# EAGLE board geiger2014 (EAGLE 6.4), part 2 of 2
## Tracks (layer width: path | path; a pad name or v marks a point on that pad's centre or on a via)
N$1  (via drill 0.6)
  Top 0.406: v139.7,58.17 138.68,58.29 121.79,58.29 114.3,65.66 95.89,65.66 95.89,67.82 73.15,67.82 73.15,60.07 72.64,59.82 69.47,59.82 68.2,61.72 v55.24,61.72 | v55.24,56.26 55.24,30.61 54.61,29.97 33.27,29.97
  Top 0.61: v17.78,29.97 v21.97,29.97 33.27,29.97
  Top 0.813: v139.7,58.17 143,58.17 143,53.09 143.26,52.83 156.97,52.83 159.26,52.83 161.54,50.55 v161.42,50.44
  Top 1.016: v146.05,75.95 v146.05,74.93 v146.05,73.91 146.05,67.94 158.5,67.94 158.5,66.04 159.77,64.77 159.77,60.45 156.97,57.66 156.97,52.83
  Bottom 0.61: IC5.7 178.31,50.04 177.04,51.31 176.02,51.56 175.81,51.78 C19.+ | IC2.14 18.41,6.73 20.45,8.26 20.45,15.37 21.97,17.4 v21.97,29.97 | v17.78,29.97 T1.3 | v55.24,56.26 v55.24,61.72
  Bottom 0.813: IC4.14 160.02,49.02 160.02,50.44 v161.42,50.44 163.35,50.44 163.32,50.42 163.32,52.83 165.61,55.12 171.25,55.12 R38.1 174.23,54.91 C19.+ | Q4.3 v139.7,58.17
  Bottom 1.016: C13.1 147.06,79.5 147.32,79.25 147.32,78.34 L1.2 147.81,75.95 v146.05,75.95 v146.05,74.93 v146.05,73.91
N$2
  Bottom 1.016: 139.83,69.72 139.83,70.48 137.54,72.77 125.48,72.77
N$3  (via drill 0.6)
  other vias: 89.15,18.29
N$4
  Top 0.406: X1.1 213.94,43 212.34,41.4 212.34,35.28 J1.2
  Bottom 1.27: F1.2 200.91,30.35 200.91,34.8 201.27,35.15 J1.2 212.57,34.8 215.14,34.8 215.22,34.72 J1.3
N$5  (via drill 1.2 pad 2.54)
  Bottom 0.406: 194.82,74.17 196.34,74.17
  Bottom 0.813: 194.82,74.17 197.87,74.17 199.14,72.9 199.14,66.55 198.63,66.04 198.63,62.99 199.9,61.72 199.9,45.21 202.18,42.93 202.18,41.4 202.44,41.15
  Bottom 1.27: v201.42,41.15 202.44,41.15 v203.84,41.15 | v203.84,41.15 v206.25,41.15 | 203.71,41.27 v203.84,41.15
N$6
  Bottom 0.61: R5.1 13.01,26.74 T1.1
N$7
  Bottom 0.813: D7.C D6.A 170.86,74.09 C6.1 C4.2
N$8
  Bottom 0.305: C11.2 188.6,19.43 188.59,19.3 183.9,19.3 183.39,19.81 181.1,19.81 181.1,15.75 180.59,15.24 179.96,15.24 179.07,14.48 179.07,10.92 179.71,10.41 180.85,10.41 | 180.85,10.41 182.25,10.41 182.25,11.91 185.76,11.91 185.76,11.85 | R57.1 180.85,10.41
  Bottom 0.406: IC3.6 187.07,10.79 185.76,11.85
N$9
  Bottom 0.406: R9.2 177.42,17.83 177.42,17.65 178.82,16.26 179.94,16.26 T3.1
N$10
  Bottom 0.61: R12.2 175.08,30.73 175.9,30.73 176.28,30.99 176.78,31.75 182.37,31.75 182.37,28.19 182.5,27.69 182.5,21.34 183.51,20.95 C11.1
N$11
  Bottom 0.406: 203.2,18.8 203.45,18.54
N$12  (via drill 0.6)
  Top 0.406: v137.92,43.18 136.78,44.45 135.25,44.96 135.25,54.36 122.94,54.36 121.16,55.63 119.38,55.63 113.28,61.72 101.35,61.72 101.35,62.48 100.84,62.99 95.25,62.99 91.06,63.75 85.47,63.75 83.82,65.28 76.58,65.28 v76.58,56.52
  Bottom 0.406: v76.58,56.52 77.98,57.55 IC7.34 | 175.01,18.36 175.01,18.41 175.01,23.88 | 175.01,18.49 175.21,18.29 175.46,18.29 R9.1
  Bottom 0.61: R11.1 R10.1 175.26,23.88 175.01,24.13 | 175.01,24.13 175.01,23.88 175.01,18.59 | 175.01,24.13 164.72,24.13 164.72,36.32 146.05,36.32 140.72,41.66 139.45,41.66 v137.92,43.18
  Bottom 0.813: 175.01,18.41 175.01,18.49
  Bottom 1.016: 175.01,18.41 174.12,18.41 172.59,16.89 172.59,10.92 175.51,8 T2.1
N$13
  Bottom 0.813: Q10.C 114.74,41.47 115.19,41.02 116.08,39.88 116.08,38.81 R50.1
N$14
  Bottom 0.406: DIS1.16 48.97,34.54 Q6.C
N$15
  Bottom 0.61: IC3.3 187.07,12.83 188.09,11.56 192.91,11.56 193.93,12.85 194.49,14.05 | 194.49,14.05 194.74,14.3 | IC1.1 196.17,12.36 194.49,14.05
  Bottom 1.016: R7.1 194.74,14.3 194.31,14.48 194.31,19.56 193.8,20.07 193.04,20.83 C8.1
N$16  (via drill 0.6, 0.6 pad 1.68)
  Top 0.406: v190.5,26.42 190.5,22.61 186.18,22.61 185.93,22.35 v185.93,16.51 185.93,6.99 v182.25,6.99
  Bottom 0.406: R17.2 R20.2 R21.2 | IC3.2 185.93,14.63 v185.93,16.51 | v190.5,26.42 188.14,26.42 | R21.2 170.49,34.29 175.01,34.29 | R24.2 170.61,31.62 R23.2 R21.2 | v175.01,35.56 175.01,34.04
  Bottom 0.61: R13.1 188.14,26.42 188.14,25.58 187.96,25.4 186.18,25.4 186.18,23.8 R14.2 186,23.88 184.66,23.88 184.15,24.38 184.15,33.53 182.88,34.29 175.01,34.29 175.01,34.04 R12.1 | R24.2 R26.2
N$17
  Bottom 1.016: 124.84,67.56 124.97,67.69
N$18
  Bottom 0.61: Q4.1 140.64,51.1 R39.2 140.21,49.61 140.21,47.5 138.81,47.5 138.75,47.31 Q5.C
N$19
  Bottom 0.406: R53.2 150.04,5.21 147.19,5.21 146.9,5.12 Q12.2 146.9,5.04 146.43,3.94 144.02,3.94 143.89,4.7 143.89,4.83 142.37,6.35 127,6.35 K1.7
  Bottom 1.016: K1.7 121.28,4.32 121.28,12.57 | 121.28,12.57 121.28,16.51 122.43,17.65 123.66,17.65 S1.4 | 121.28,12.57 121.16,12.7 114.94,12.7 114.17,13.46 C30.1 109.85,13.46 108.46,14.1 98.68,14.1 98.68,13.21 89.92,13.21 89.92,11.68 81.53,11.68 81.53,5.33 SL1.4
  Bottom 1.27: S1.3 S1.4
N$20  (via drill 0.6)
  Top 0.406: v107.19,45.72 91.31,45.72 v91.31,48.51 | v99.57,68.45 99.57,70.87 86.87,70.87 86.49,69.34 70.61,69.34 v70.61,70.48
  Bottom 0.406: IC7.1 79.82,71.37 | 79.82,71.37 79.82,75.38 PR1.1 | Q10.B 112.15,45.72 v107.19,45.72 | v91.31,48.51 91.31,53.34 92.2,53.34 94.23,54.61 94.23,57.78 99.06,57.78 99.57,58.17 v99.57,68.45 | v70.61,70.48 70.61,71.12 70.99,71.5 79.69,71.5 79.82,71.37
N$21  (via drill 1.2 pad 2.54)
  Bottom 1.016: v205.99,64.77 v203.71,64.77 v201.42,64.77
N$22
  Bottom 0.61: Q12.1 147.07,7.98 147.07,9.02 147.57,9.53 150.24,9.53 | 150.24,9.53 R53.1 | Q13.C 153.42,6.67 153.42,9.27 153.29,9.53 150.24,9.53
N$23
  Bottom 0.813: 194.82,78.74 195.33,78.74 196.85,77.22 201.93,77.22 201.93,65.28 202.18,65.02 201.68,64.52
N$24  (via drill 0.6)
  Top 0.406: v166.37,28.96 162.94,32.38 162.56,34.54 161.54,35.56 143.26,35.56 140.72,38.1 134.87,38.1 133.1,39.88 119.38,39.88 115.57,43.69 115.57,50.8 115.32,50.8 109.73,56.39 94.23,56.39 94.23,54.61 v91.44,54.61
  Bottom 0.406: R26.1 166.88,28.19 v166.37,28.96 | v91.44,54.61 89.92,54.61 89.41,54.36 87.12,54.36 87.02,54.46 IC7.24
N$25  (via drill 0.6)
  Top 0.406: 123.83,22.26 S1.2 119.38,22.26 119.38,36.07 112.78,42.67 112.78,49.28 108.71,53.34 97.28,53.34 97.28,50.55 84.07,50.55 84.07,46.1 71.5,46.1 v71.5,46.48
  Bottom 0.406: IC7.36 78.01,59.18 71.5,59.18 v71.5,46.48 | D14.A 138.76,18.37 136.14,15.75 R35.1
  Bottom 0.61: S1.2 S1.1 130.34,22.35 134.24,22.35 134.24,20.07 139.45,20.07 D14.A
N$26  (via drill 0.6)
  Top 0.406: v166.37,35.05 165.74,36.07 165.1,36.7 163.96,37.59 163.32,37.85 144.02,37.85 141.48,40.39 135.64,40.39 133.86,42.16 121.41,42.16 117.86,45.72 117.86,52.58 117.35,52.58 111.25,58.67 96.52,58.67 v96.01,59.18
  Bottom 0.406: R21.1 v166.37,35.05 | v96.01,59.18 92.96,58.55 91.42,58.4 IC7.21
N$27  (via drill 0.6)
  Top 0.406: v133.6,25.91 133.6,38.1 132.59,39.12 118.87,39.12 114.81,43.18 114.81,50.04 109.47,55.37 95.25,55.37 95.25,52.32 v85.6,52.32
  Bottom 0.406: v85.6,52.32 85.42,53.67 IC7.26 | v133.6,25.91 135.84,25.91 D18.A
N$28  (via drill 0.6)
  Top 0.406: K1.5 130.05,6.22 128.27,8 96.77,8 94.74,10.03 94.74,20.19 95.25,20.7 115.06,20.7 115.19,20.57 v115.19,18.54
  Bottom 0.406: Q2.C 113.72,18.55 112.58,18.55 | 112.58,18.55 D17.A | 112.58,18.55 112.59,18.54 v115.19,18.54
N$29  (via drill 0.6)
  Top 0.406: v80.52,48.26 v80.52,51.56
  Bottom 0.406: IC7.29 83.06,55.76 82.93,53.72 81.03,52.07 v80.52,51.56 | C22.2 85.22,44.2 84.96,43.94 80.77,43.94 80.77,48.26 v80.52,48.26
N$30  (via drill 0.6)
  Top 0.406: v166.37,32.77 165.23,33.27 164.85,33.91 164.47,35.81 164.21,36.07 163.7,36.32 162.94,37.08 143.76,37.08 141.22,39.62 135.38,39.62 133.6,41.4 120.65,41.4 117.09,44.96 117.09,51.82 116.84,51.82 110.74,57.91 92.46,57.91 v91.57,57.02
  Bottom 0.406: R23.1 v166.37,32.77 | v91.57,57.02 90.81,57.02 89.98,57.59 IC7.22
N$31  (via drill 0.6)
  Top 0.406: v143.51,17.27 143.51,27.43 v175.01,27.43
  Bottom 0.406: R16.1 177.29,29.72 176.78,29.21 175.13,28.57 v175.01,27.43 | D12.A v143.51,17.27
N$32  (via drill 0.6)
  Bottom 0.813: 194.82,69.85 196.6,69.85 197.1,69.34 197.1,66.55 196.6,66.04 196.6,62.23 197.61,61.21 197.61,39.62 199.14,38.1 216.66,38.1 218.69,36.07 218.69,23.37 215.14,23.37 213.11,21.34 v213.11,18.54 213.11,18.29
N$33
  Bottom 0.61: T1.2 13.44,30.86 11.56,30.86 10.79,29.84 R6.1 9.45,24.08 10.16,23.37 14.73,23.37 16.76,21.34 16.76,16 15.49,16 13.97,14.48 13.97,8.38 14.22,8.13 15.24,8.13 15.49,7.87 16.15,7.87 IC2.13
N$34
  Bottom 0.813: 19.56,26.29 19.56,26.42
N$35  (via drill 0.6)
  Top 0.406: v145.54,22.73 145.54,23.62 145.8,23.88 154.94,23.88 v155.23,23.58
  Top 1.27: 112.78,71.63 v112.78,71.12 v112.78,69.85 v131.57,69.85 v132.84,69.85 v134.24,69.85 135,69.85
  Bottom 0.406: IC8.8 148.8,21.77 D16.C | R36.2 155.88,18.87 155.19,19.56 155.19,21.84 154.34,22.69 | R45.1 R48.1 R46.1 | R44.2 Q8.2 77.34,27.69 70.99,27.69 67.69,31.11 67.78,37.97 | IC8.5 145.56,21.86 145.54,21.84 v145.54,22.73 | R56.1 66.22,47.42 66.29,47.5
  Bottom 0.61: R39.1 138.63,51.35 Q4.2 135.72,53.51 135.64,53.59 | D15.A 84.45,17.02 84.45,19.56
  Bottom 1.016: SL1.2 76.2,19.56 84.45,19.56 84.84,19.94 84.84,34.04
  Bottom 1.27: C20.+ 158.24,25.15 156.8,25.15 | 156.8,25.15 v155.23,23.58 154.34,22.69 D16.C | C28.2 143.39,33.66 144.02,34.29 | 144.02,34.29 v149.1,34.29 155.7,34.29 155.7,25.61 156.8,25.15 | JP1.2 v112.78,71.12 v112.78,69.85 112.78,62.48 112.52,62.23 106.17,62.23 103.12,58.55 103.12,55.37 98.04,55.37 96.77,54.74 C27.1 95.37,52.32 94.49,51.69 93.98,51.31 SG1.+ 93.98,37.85 | LED1.A 107.31,42.8 107.19,42.67 107.19,38.86 105.92,37.59 94.23,37.59 93.98,37.85 | 144.02,34.29 144.02,36.07 141.73,38.35 135.89,38.35 135.64,38.61 135.64,53.59 135.64,69.34 135.13,69.85 v134.24,69.85 v132.84,69.85 v131.57,69.85 | 93.98,37.85 73.66,37.85 67.78,37.97 66.29,38.61 | 66.29,38.61 66.29,47.5 66.29,55.88 R46.1 | 66.29,38.61 66.29,34.16 66.42,34.04 84.84,34.04 104.27,34.04
N$36  (via drill 0.6)
  Top 0.406: v166.37,31.11 165.35,31.5 163.7,33.4 163.58,35.05 162.31,36.32 143.51,36.32 140.97,38.86 135.13,38.86 133.35,40.64 119.89,40.64 116.33,44.2 116.33,51.31 116.08,51.31 110.24,57.15 93.73,57.15 93.22,56.64 v92.96,55.88
  Bottom 0.406: R24.1 167.13,30.48 v166.37,31.11 | v92.96,55.88 93.13,55.8 IC7.23
N$37  (via drill 0.6)
  Top 0.406: v91.31,68.83 96.9,68.83 96.9,66.42 102.23,66.42 102.49,66.67 102.62,67.06 102.74,67.18 v104.27,67.18 | v68.33,40.01 59.18,40.01 v59.18,38.23
  Bottom 0.406: IC7.10 87,68.83 87.63,69.34 90.3,69.34 v91.31,68.83 | v104.27,67.18 104.27,63.25 101.35,60.2 101.35,56.9 101.22,56.77 95.25,56.77 95.12,56.64 95.12,54.1 92.46,52.32 92.46,44.45 91.69,43.81 91.19,43.43 91.19,39.5 69.85,39.5 v68.33,40.01 | v59.18,38.23 Q6.B
N$38
  Top 0.406: 213.36,18.54 205.74,18.54
N$39
  Bottom 0.61: IC2.12 IC2.11
N$40  (via drill 0.6)
  Top 0.406: v165.1,40.39 164.72,40.39 164.34,39.88 163.83,39.37 144.53,39.37 141.99,41.91 136.14,41.91 134.37,43.69 122.43,43.69 119.38,46.74 119.38,54.1 118.36,54.1 112.27,60.2 99.82,60.2 99.31,60.71 99.31,61.21 v93.73,61.21
  Bottom 0.406: R17.1 167.39,39.62 166.12,40.39 v165.1,40.39 | v93.73,61.21 92.46,60.96 90.42,59.94 89.67,59.94 IC7.19
N$41
  Bottom 0.813: D2.C D1.A 187.37,74.09 C2.1
N$42
  Bottom 0.813: R4.1 11.66,33.02 14.22,32.77 14.48,32.51 19.56,32.51 19.56,26.42 R5.2
N$43
  Bottom 0.813: D4.C D3.A 179.58,74.09 179.58,78.23 179.12,78.23 C4.1 C2.2
N$47
  Bottom 0.813: C10.2 155.21,78.11 L1.1 155.57,77.85 D10.A
  Bottom 1.016: T4.2 T4.4 149.22,68.78 149.22,73.91 149.27,74.09 D10.A
N$48
  Bottom 0.61: R18.1 R22.2
N$49
  Bottom 0.813: C1.2 C3.1 180.34,66.67 180.34,70.69 | D2.A 180.34,70.69 | 180.34,70.69 D3.C
N$50
  Bottom 0.813: R2.1 R1.1 R3.1 188.47,69.85 | C1.1 188.47,66.67 188.47,69.85 | 188.47,69.85 188.47,70.61 187.32,70.61 D1.C
N$51  (via drill 0.6)
  Top 0.406: v145.29,62.48 v145.29,55.37
  Bottom 0.406: IC4.2 155.07,46.1 154.94,46.23 152.4,46.23 | 152.4,46.23 152.4,43.03 IC4.4 | 152.4,46.23 151.64,46.23 151.26,46.61 IC4.10 151.13,49.17 151.13,51.05 | T4.1 143.53,64.49 145.29,62.74 v145.29,62.48 | IC4.12 153.8,50.93 153.67,51.05 151.13,51.05 | v145.29,55.37 145.29,54.86 | 145.29,54.86 145.29,50.55 145.82,50.32 IC4.8 | 151.13,51.05 150.37,51.82 150.37,54.1 149.61,54.86 145.29,54.86
N$52
  Bottom 0.61: R22.1 R25.2
N$53
  Bottom 0.813: D4.A 176.23,70.69 C3.2 C7.1 172.21,66.67 172.21,70.61 171.45,70.61 D6.C
N$54
  Bottom 0.406: R47.1 103.38,49.61
  Bottom 0.61: 103.38,49.61 103.38,43.18 101.6,41.4 SG1.-
N$55
  Bottom 0.61: R25.1 R27.2
N$56
  Bottom 0.813: D8.C D7.A 167.64,66.67 | C7.2 167.64,66.67 | 167.64,66.67 C9.1
N$57
  Bottom 0.61: R27.1 R29.2
N$58
  Bottom 0.813: C6.2 C10.1 163.19,78.11 D8.A D9.C
N$59
  Bottom 0.61: R18.2 183.13,60.63 183.13,62.87 183.13,62.99 163.07,62.99 162.31,64.01 160.78,64.01 159.77,65.02 160.02,66.47 C9.2
  Bottom 0.813: C12.1 155.57,66.67 D10.C D9.A 160.23,70.69 C9.2
N$60  (via drill 0.6)
  Top 0.406: v114.55,72.9 110.49,72.9 109.09,71.75 86.11,71.75 85.72,70.1 77.47,70.1 77.47,71.75 68.58,71.75 68.58,65.66 68.71,65.53 | v70.99,62.48 70.99,65.53 68.71,65.53 | 53.85,52.7 53.85,62.99 63.12,62.99 63.63,63.12 63.63,65.53 68.71,65.53
  Top 0.61: v18.8,16.64 20.57,16.64 22.48,19.3 22.48,26.16 21.21,27.43 15.24,27.43 15.24,31.88 32.77,31.88 53.85,52.7
  Bottom 0.305: R58.2 115.32,72.9 v114.55,72.9
  Bottom 0.406: v70.99,62.48 75.69,62.48 76.45,63.25 77.97,63.25 IC7.41
  Bottom 0.61: IC2.10 18.54,11.81 18.8,12.06 v18.8,16.64
N$61
  Bottom 0.61: R29.1 R31.2
N$62  (via drill 0.6)
  Top 0.406: v156.46,63.25 147.57,63.25 145.54,65.28 138.18,65.28 138.18,74.93 R34.E
  Bottom 0.406: R34.S 127.76,74.93 R34.E | R31.1 164.85,60.63 | 164.85,60.63 163.14,60.63 161.04,62.74 156.72,62.74 | 156.72,62.74 C17.1 | IC5.2 178.31,44.96 179.07,45.72 180.85,45.72 181.36,46.48 181.36,50.04 180.09,51.31 179.32,51.31 178.31,52.32 178.31,55.63 177.8,56.13 173.48,56.13 172.72,56.9 164.85,56.9 164.85,60.63 | 156.72,62.74 156.46,62.99 v156.46,63.25
N$63
  Bottom 0.406: D18.C 139.24,25.96 137.79,24.51 132.08,24.51 132.08,26.92 130.58,26.92 Q1.1 130.51,28.15 130.56,28.19 125.22,28.19 C33.1 124.21,28.07 123.95,28.32 118.75,28.32 118.62,28.19 118.62,26.47 R52.1
N$64
  Bottom 0.406: D13.C 149.1,52.27 149.1,51.56 149.86,50.8 149.86,50.04 150.11,49.78 150.11,49.17 IC4.9 IC4.6 149.99,41.02 150.11,40.89 153.92,40.89 | 153.92,40.89 153.92,42.77 IC4.3 | 153.92,40.89 156.21,40.89 156.34,41.02 IC4.1 156.46,45.72 155.96,47.12 155.83,47.24 154.69,47.24 | IC4.13 155.07,47.62 154.69,47.24 | 154.69,47.24 152.91,47.24 152.65,47.5 | 152.65,47.5 152.65,48.92 IC4.11 152.53,47.62 152.65,47.5
N$65
  Bottom 0.406: D13.A 154.51,52.83 R30.2
N$66  (via drill 0.6)
  Top 0.406: v158.24,50.8 158.24,45.97 151.38,45.97 v151.38,44.7
  Bottom 0.406: C16.2 150.11,60.45 150.11,59.18 150.57,58.73 R32.2 150.62,56.46 151.89,54.86 156.46,54.86 156.51,54.3 R30.1 158.24,50.98 v158.24,50.8 | v151.38,44.7 151.26,44.58 IC4.5
N$67
  Bottom 0.61: Q9.C 105.16,56.32 105.16,51.82 105.11,51.61 R47.2
N$68
  Bottom 0.406: 197.1,80.77 191.52,80.77 191.52,78.99 191.64,78.99 191.64,78.74
N$69
  Bottom 0.61: IC6.1 169.14,48.77 171.7,48.77 | 171.7,48.77 171.83,48.64 C18.1 172.84,46.61 174.24,45.21 176.53,45.21 177.04,44.7 IC5.3 | R38.2 171.7,52.78 171.7,48.77
N$70
  Bottom 0.813: 7.11,18.54 7.24,18.54
  Bottom 1.016: 12.83,18.54 7.24,18.54
N$71  (via drill 0.6)
  Top 0.406: v141.99,11.18 99.19,11.18 v99.19,17.02 99.19,17.14
  Bottom 0.406: v141.99,11.18 R42.1 | v99.19,17.02 97.16,16.97 D15.C
N$72  (via drill 0.6)
  Top 0.406: v174.24,50.29 173.48,51.05 173.48,53.59 172.97,54.36 v160.02,54.36
  Bottom 0.406: R32.1 152.83,56.9 R33.1 160.1,54.18 v160.02,54.36 | IC5.6 177.04,49.78 176.53,50.29 v174.24,50.29
N$73
  Bottom 0.406: R54.1 82.63,16.76 D20.A 82.68,14.81 82.68,12.95 87.76,12.95 87.76,14.48 96.39,14.48 96.65,15.11 96.77,15.24 106.68,15.24 106.81,15.49 106.81,19.18 111,19.18 111.51,20.07 111.51,25.21 Q2.B
N$74
  Bottom 0.61: C17.2 160.4,59.44 161.04,58.93 161.98,57.99 R33.2
N$75
  Bottom 0.406: 148.97,17.4 149.99,16.64 149.99,13.84
N$76
  Bottom 0.61: R34.A 137.67,80.01 137.67,78.92 R37.1
N$77
  Bottom 0.406: D16.A 153.42,18.54 | 152.53,18.54 151.38,20.57 148.08,20.57 148.08,21.86 | L2.2 153.06,24.38 148.08,24.38 148.08,21.86 | 148.08,21.86 IC8.7
  Bottom 0.813: 153.42,18.54 152.53,18.54
N$78
  Bottom 0.406: 149.1,17.65 150.37,16.76 150.37,13.84
N$79
  Bottom 0.406: IC8.4 146.3,16.96 146.3,13.21 C24.1
N$80  (via drill 0.6)
  Top 0.406: v108.2,25.15 108.2,31.75 118.24,31.75 118.24,35.43 115.7,37.97 108.71,37.97 108.71,49.78 87.88,49.78 v87.88,49.02
  Bottom 0.406: 108.27,25.21 v108.2,25.15 108.2,20.45 96.14,20.45 95.12,18.8 95.12,15.62 94.87,15.37 86.03,15.37 | v87.88,49.02 87.88,52.32 86.23,53.98 86.23,55.55 IC7.25 | 85.98,15.37 86.03,15.37 | 86.11,15.37 86.03,15.37 | 86.03,15.37 D20.C
N$81
  Bottom 0.406: 149.1,19.56 149.1,17.78
N$82  (via drill 0.6)
  Top 0.406: TR1.1 159.26,14.61 140.08,14.61 140.08,15.24 119.76,15.24 116.2,21.59 75.56,21.59 75.56,34.16 71.75,34.16 v71.75,44.7
  Bottom 0.406: 160.02,20.83 157.43,20.83 R36.1 | R36.1 160.02,20.75 160.02,20.83 | 160.02,20.83 160.53,20.45 | 160.53,20.45 161.8,19.05 TR1.1 | R36.1 160.15,20.75 160.53,20.45 | 160.53,20.45 162.18,18.8 | IC7.37 77.97,59.94 70.74,59.94 70.36,59.56 70.36,44.83 70.48,44.7 v71.75,44.7
N$83
  Bottom 0.406: 149.35,19.3 149.35,17.65
N$84  (via drill 0.6)
  Top 0.406: S2.3 96.29,75.46 95.63,74.8 88.27,74.8 88.27,75.44 | 88.27,75.44 88.27,76.83 PR1.5 | 88.27,75.44 83.19,75.44 82.42,74.68 82.42,71.37 v82.68,71.12
  Bottom 0.406: R40.2 101.73,70.48 101.73,75.46 | v82.68,71.12 82.68,70.23 82.3,69.85 82.3,67.47 IC7.4
  Bottom 1.27: S2.4 101.73,75.46 S2.3
N$85
  Bottom 0.406: IC7.27 84.58,55.76 84.58,54.36 84.2,51.56 84.71,50.92 C25.2 87,47.88 87,43.69 86.49,42.93 79.38,42.93 78.58,43.72 L3.2
N$86
  Bottom 0.813: LED1.K 110.49,39.88 111.76,38.61 113.74,38.61 R50.2
N$87
  Bottom 0.406: 149.1,21.97 152.53,21.97
N$88  (via drill 1.2 pad 2.54)
  Bottom 1.27: v201.42,18.41 v205.87,18.41
N$89  (via drill 0.6)
  Top 0.406: S4.3 130.3,59.69 130.18,61.98 120.78,61.98 115.19,67.18 110.62,67.18 110.62,69.09 101.35,69.09 101.35,67.31 98.17,67.31 98.17,69.98 87.76,69.98 87.12,68.58 72.26,68.58 72.26,60.96 70.1,60.96 69.85,61.21 v69.85,64.14
  Bottom 0.406: R46.2 v69.85,64.14 75.82,64.14 75.95,64.01 78.01,64.01 IC7.42
N$90  (via drill 0.6)
  Top 0.406: S5.3 128.24,47.75 120.27,47.75 120.27,54.61 119.89,54.86 118.87,54.86 112.78,60.96 100.33,60.96 100.33,61.98 100.08,62.23 94.87,62.23 91.06,62.99 84.45,62.99 83.57,64.26 v81.66,64.26
  Bottom 0.406: R48.2 74.68,66.8 76.71,64.77 78,64.77 IC7.43 78.05,64.77 79.76,64.77 79.88,64.26 v81.66,64.26
N$91
  Bottom 0.406: 152.78,28.07 152.78,24.64
N$92  (via drill 0.6)
  Top 0.406: v107.44,77.47 93.47,77.47 93.22,77.22 PR1.9
  Bottom 0.406: IC7.2 80.62,72.49 80.64,73.03 93.22,73.03 PR1.9 | Q7.B 115.57,56.78 115.57,59.69 117.47,62.99 117.47,75.31 115.06,77.47 v107.44,77.47
N$93
  Bottom 0.406: 148.34,24.13 153.03,24.13
N$94
  Bottom 0.61: DIS1.15 19.12,37.08 18.67,37.08 R43.1
N$95  (via drill 0.6)
  Top 0.406: v87.38,61.72 87.38,54.1 87.12,53.72 80.52,53.72 78.99,52.45 59.82,52.45 v59.56,52.2
  Bottom 0.406: IC7.16 88.18,62.4 88.14,62.36 88.01,62.36 v87.38,61.72 | v59.56,52.2 40.01,52.2 27.56,39.75 24,39.75 DIS1.14
N$96  (via drill 0.6)
  Top 0.406: v86.23,59.05 86.23,54.86 86.11,54.61 80.26,54.61 78.61,53.34 60.83,53.34 60.33,53.59 v58.42,53.59
  Bottom 0.406: IC7.15 86.82,63.2 86.49,62.87 86.23,62.36 v86.23,59.05 | v58.42,53.59 39.5,53.59 38.99,53.34 27.81,42.29 24,42.29 DIS1.13
N$97
  Bottom 0.813: R49.S 66.29,77.22 61.72,77.22 59.69,75.18 51.56,75.18 43.94,67.56 DIS1.3
N$98  (via drill 0.6)
  Top 0.406: v84.96,60.58 84.96,60.07 83.82,58.42 83.82,56.39 79.76,56.39 79.76,55.37 78.36,54.23 61.21,54.23 v59.94,55.24
  Bottom 0.406: IC7.14 85.61,63.99 85.6,64.01 84.96,63.37 v84.96,60.58 | v59.94,55.24 59.69,55.24 56.39,54.48 38.23,54.48 30.61,46.99 28.32,44.83 DIS1.12
N$99
  Bottom 0.406: 148.97,22.23 152.78,22.23
N$100  (via drill 0.6)
  Top 0.406: 50.54,59.94 51.3,59.94 v51.18,59.94 | v59.56,59.31 68.33,59.31 69.22,58.42 72.77,58.42 73.79,59.31 74.04,59.56 74.04,66.8 74.17,66.93 89.32,66.93 89.62,66.63 90.76,66.63 v90.81,66.67
  Top 0.61: DIS1.6 50.54,59.94 50.55,59.94
  Bottom 0.406: IC7.12 89.62,66.63 v90.81,66.67 | v51.18,59.94 51.18,63.37 59.56,63.37 v59.56,59.31
N$101  (via drill 0.6)
  Top 0.406: v87.12,65.28 87.12,65.66 86.87,66.04 75.06,66.04 75.06,58.42 73.79,57.15 v63.63,57.15 | 50.55,65.02 59.82,65.02 60.07,65.28 60.07,68.2 v63.5,68.2
  Top 0.61: DIS1.4 50.54,65.02 50.55,65.02
  Bottom 0.406: IC7.11 87.88,67.39 87.88,65.79 v87.12,65.28 | v63.5,68.2 63.5,56.9 v63.63,57.15
N$102  (via drill 0.6)
  Top 0.406: S3.3 127,34.99 127,37.85 126.75,38.1 118.62,38.1 114.05,42.67 114.05,49.53 109.22,54.36 96.27,54.36 96.27,51.31 82.3,51.31 82.3,47.12 77.22,47.12 77.22,50.42 v64.39,50.42
  Bottom 0.406: IC7.44 77.41,65.59 74.17,68.58 69.98,68.58 69.22,69.6 R45.2 68.25,71.45 67.94,71.5 64.77,71.5 64.77,62.61 65.02,62.36 65.02,55.63 64.9,55.63 64.52,55.5 64.52,50.55 v64.39,50.42
N$103
  Bottom 0.406: 142.49,24.89 142.49,24.26 142.62,24.13 147.19,24.13 147.19,23.11
N$104  (via drill 0.6)
  Top 0.406: v96.01,81.03 81.03,81.03 80.26,80.26 79.63,79.76 79.25,79.5 79.25,72.64 65.28,72.64 65.15,72.52 65.15,66.93 64.77,66.55 61.34,66.55 61.21,66.42 61.21,64.01 52.58,64.01 52.58,57.28 50.42,57.28
  Top 0.61: DIS1.11 37.08,47.24 36.45,47.24 39.75,47.24 50.42,57.28
  Bottom 0.406: IC7.13 91.67,64.8 91.69,64.77 96.39,64.77 96.39,80.64 v96.01,81.03
N$107
  Bottom 1.27: 208.91,14.1 216.41,14.1
N$108
  Bottom 0.406: 202.18,18.29 205.49,18.29
N$109  (via drill 0.6 pad 2.18)
  other vias: 197.61,80.77
N$110  (via drill 0.6)
  Bottom 1.016: 93.22,27.05 92.84,27.05 92.84,19.56 91.57,18.29 v86.36,18.29
N$111  (via drill 1.2 pad 2.54)
  other vias: 12.45,18.67
N$112  (via drill 0.6, 1.2 pad 2.54)
  Top 0.61: v2.03,32 v9.27,32
  Bottom 0.61: 11.56,33.27 10.29,32 v9.27,32
  Bottom 1.27: v7.37,18.67 2.67,18.67 2.67,19.05 2.03,20.07 v2.03,32 2.03,40.13 3.05,41.15 6.86,41.15 7.11,41.4 7.37,41.4
N$113  (via drill 1.2 pad 2.54)
  other vias: 12.45,41.4
N$114  (via drill 1.2 pad 2.54)
  Bottom 1.27: v7.37,41.4 v9.91,41.4
N$115  (via drill 1.2 pad 2.54)
  other vias: 12.45,64.39
N$116  (via drill 1.2 pad 2.54)
  Bottom 0.406: v9.91,64.39 v7.37,64.39
N$117  (via drill 0.6)
  Top 0.406: v165.1,38.61 144.27,38.61 141.73,41.15 135.89,41.15 134.11,42.93 121.92,42.93 118.62,46.23 118.62,53.34 117.86,53.34 111.76,59.44 99.06,59.44 v98.04,60.07
  Bottom 0.406: R20.1 167.51,37.21 v165.1,38.61 | v98.04,60.07 97.79,60.45 95.5,60.45 94.36,59.94 92.96,59.94 91.19,59.18 90.17,59.18 90.16,59.2 IC7.20
N$118
  Bottom 0.813: 12.45,41.02 12.45,41.53 9.91,41.53 7.24,41.53 7.24,41.4 7.37,41.4 | 12.32,64.64 12.32,64.39
  Bottom 1.016: 7.37,64.64 12.32,64.64
  Bottom 1.27: 12.32,64.39 9.91,64.39 9.91,41.53
N$119
  Bottom 0.406: D19.C R54.2
N$120
  Bottom 1.27: 66.93,25.91 62.1,28.7
N$121  (via drill 1.2 pad 2.54)
  other vias: 203.58,18.41
N$122  (via drill 0.6)
  Top 1.016: 73.53,5.21 73.66,5.21 73.66,18.29 v90.55,18.29
N$123  (via drill 0.6)
  other vias: 87.76,18.29
N$124
  Bottom 1.27: 67.31,37.72 67.31,34.8
N$126
  Bottom 0.406: 194.82,78.49 194.56,78.74
N$127  (via drill 1.2 pad 2.54)
  other vias: 9.91,18.67
N$128  (via drill 0.6 pad 2.54)
  other vias: 216.53,13.97
N$129  (via drill 0.6)
  Bottom 0.305: 78.61,62.36 80.64,62.36 v80.64,62.74 80.64,62.87
N$131  (via drill 0.6)
  Top 0.406: v171.32,22.48 182.5,22.48 182.5,30.1 192.79,30.1 192.79,21.59 v189.87,18.67
  Bottom 0.305: 181.95,14.9 181.95,14.87 R57.2
  Bottom 0.406: R8.1 190.45,17.2 189.74,18.54 | 189.74,18.54 182.88,18.54 182.5,17.27 182.37,17.44 T3.3 181.95,17.02 181.95,14.9 | T2.3 172.59,3.43 171.2,4.83 171.2,22.35 v171.32,22.48 | v189.87,18.67 189.74,18.54
N$135
  Bottom 0.305: R58.1 115.32,62.1 112.9,59.69 112.9,57.72 Q7.C
  Bottom 0.61: Q7.C 112.53,57.34 Q9.B
N$136  (via drill 0.6)
  Top 0.406: v139.45,23.62 141.48,23.62 141.48,16.26 142.11,15.75 v144.53,15.75
  Bottom 0.406: D14.C v139.45,23.62 | v144.53,15.75 143.18,15.24 R42.2 | D11.C 136.02,21.77 136.02,23.62 124.97,23.62 124.97,24.64 126.28,25.91 Q1.3
  Bottom 0.61: D12.C 139.32,22.15 D14.C D11.C | R42.2 142.24,15.24 141.73,15.75 139.78,15.75 R41.1 | Q13.B 155.57,7.87 155.57,10.67 155.19,11.05 144.53,11.05 v144.53,15.75
N$137  (via drill 0.6)
  Top 0.406: v191.26,8.64 191.26,10.16 195.07,13.46 195.83,14.22 v195.83,21.59 | v120.65,33.4 120.65,24.51 v123.06,24.51 | X1.4 215.59,45.4 214.12,46.86 210.31,46.86 210.19,46.61 210.19,38.48 208.15,36.45 208.15,31.32 J1.1
  Top 1.27: v88.77,41.27 88.77,35.43 114.3,35.43 v114.3,33.27 | 114.43,33.27 v115.44,33.27 v116.59,33.27
  Bottom 0.406: 83.82,57.78 83.82,60.71 83.78,60.54 83.82,60.88 83.82,61.72 | 83.82,57.78 IC7.28 83.82,53.85 C25.1 C22.1 | IC7.6 83.82,61.72 | IC7.39 83.69,61.59 83.82,61.72 | IC7.18 88.23,60.8 88.01,60.58 87.88,60.33 87.88,58.17 87.63,57.91 83.95,57.91 83.82,57.78 | C26.1 78.74,50.04 78.36,49.91 | C16.1 152.78,66.12 C12.2 | C24.2 149.74,16.63 149.1,17.02 149.1,17.21 IC8.1 148.84,17.51 148.84,19.56 | IC3.4 188.37,14.48 188.34,13.21 190.25,12.7 191.9,12.7 192.79,13.97 192.79,18.8 191.26,20.32 191.26,23.75 | 147.57,19.56 147.5,19.81 IC8.6 147.5,24.38 142.75,24.38 142.75,25.4 C23.2 | 147.57,19.56 148.84,19.56 | IC1.2 195.22,8.64 v191.26,8.64 | v195.83,21.59 195.58,22.61 194.56,23.62 193.55,23.62 C8.2 | PR1.10 PR1.8 PR1.6 PR1.4 85.6,80.26 84.33,81.53 78.61,81.53 78.61,74.93 75.69,74.93 | 71.75,74.93 71.63,74.93 R49.E | 147.57,19.56 146.3,19.56 145.29,20.57 141.48,20.57 141.48,17.53 140.97,17.02 138.94,17.02 137.92,16 137.92,13.08 | Q11.2 75.17,23.11 73.91,23.11 73.95,23.07 67.64,23.07 67.61,23.23 | 148.84,19.56 149.61,19.56 149.61,17.4 | DIS1.10 25.53,49.78 25.65,49.78 25.65,52.32 DIS1.9 25.65,52.32 25.65,55.12 23.87,55.12 DIS1.8 25.65,54.86 25.65,57.4 DIS1.7 21.46,57.4 21.34,57.4 21.34,62.48 | 137.92,13.08 137.92,10.41 136.02,10.41 | 136.02,10.41 133.1,10.41 | 133.1,10.41 R15.1 | R35.2 136.14,10.54 136.02,10.41 | R41.2 138.1,12.9 137.92,13.08 | C31.2 132.97,10.54 133.1,10.41 | C33.2 121.41,24.51 | 121.41,24.51 v123.06,24.51 | R28.2 111.05,32.82 111.25,33.02 | R52.2 121.16,24.46 121.16,24.51 121.41,24.51 | R55.2 61.8,36.4 61.72,36.32
  Bottom 0.61: C25.1 78.36,49.91 78.74,50.42 78.11,50.04 78.11,48.26 76.71,45.85 76.71,41.27 v88.77,41.27 | R37.2 142.8,76.91 C13.2 | IC6.2 166.88,49.13 166.88,46.23 | R4.2 7.26,30.15 R6.2 | Q5.E 142.05,44.01 143.51,42.67 146.81,42.67 | 139.32,13.41 R41.2 | C27.2 98.3,51.94 98.3,39.12 103.89,39.12 105.16,40.51 105.16,47.37 105.48,47.43 Q10.E 111.83,47.94 111.83,50.8 Q7.E 111.58,55.44 Q9.E | Q6.E 61.72,33.53 | 155.96,1.14 155.96,4.57 155.89,4.64 Q13.E
  Bottom 0.813: C18.2 171.83,42.29 171.96,42.16 175.67,42.16 IC5.4 175.51,42.01 175.51,39.62 176.02,39.12 181.1,39.12 182.88,40.13 182.88,51.31 180.81,52.62 C19.- | DIS1.1 23.87,72.9 18.54,78.23 14.35,78.23 C29.2 | 67.44,7.24 21.84,7.11 16,1.27 3.05,1.27 2.79,1.52 2.79,5.84 6.6,9.65 6.6,13.97 7.11,14.48 9.91,14.48 10.03,14.35 IC2.7 11.94,14.35 15.37,17.78 15.37,20.07 13.97,21.59 7.87,21.59 7.37,22.1 7.37,29.64 R6.2
  Bottom 1.016: C13.2 143,72.14 | 143,72.14 142.75,72.14 140.46,69.85 140.46,69.16 T4.3 | IC4.7 147.34,42.9 147.32,42.93 | 147.32,42.93 146.81,42.67 146.81,38.61 147.57,38.35 159,38.35 166.88,46.23 169.42,43.69 171.71,43.69 C18.2 | D5.2 202.22,24.86 199.64,27.43 199.39,27.43 198.37,28.45 198.37,35.31 193.42,35.31 | 193.42,35.31 189.48,35.31 | 189.48,35.31 185.93,35.31 181.1,38.61 181.1,39.12 | 193.42,35.31 C8.2 192.91,23.62 192.79,23.75 191.26,23.75 R14.1 | C15.2 189.49,33.53 189.48,35.31 | R4.2 7.26,37.49 7.37,37.59 12.95,37.59 13.08,37.72 14.99,39.88 14.99,60.45 17.02,62.48 | 17.02,62.48 21.34,62.48 DIS1.5 18.04,62.48 17.02,62.48 | 17.02,62.48 17.02,68.58 14.48,68.58 11.43,72.14 11.43,78.49 14.1,78.49 C29.2 | 143,72.14 140.21,69.34 137.67,69.34 137.67,60.45 142.49,60.45 142.75,60.2 142.75,49.78 146.81,48.01 146.81,43.69 147.32,42.93 | 118.11,36.45 111.25,36.45 111.25,33.02 111.25,27.18 Q2.E 92.72,27.05 | 118.11,36.45 118.36,36.58 118.36,49.02 | 118.36,49.02 117.47,50.16 116.84,50.8 | 116.84,50.8 111.83,50.8 | C32.2 75.69,74.93 71.75,74.93 | 118.11,36.45 118.24,36.07 118.36,49.02 | 118.36,49.02 116.84,50.8 | 116.84,50.8 118.36,52.32 118.36,58.93 120.14,60.71 120.14,67.31 120.52,67.69 125.22,67.69 | C21.- 114.05,6.52 | 114.05,6.52 114.03,6.5 C30.2 | 114.05,6.52 114.05,1.27 | C14.- 106.38,11.85 106.81,11.43 106.81,1.27
  Bottom 1.27: S2.1 S2.2 107.06,79.98 107.06,81.28 125.2,81.25 125.22,79.76 125.22,67.69 125.22,66.8 130.3,66.8 130.3,64.31 S4.1 133.1,64.26 133.1,64.01 133.1,50.04 | 133.1,36.07 138.68,36.07 139.06,35.69 C28.1 139.06,31.24 140.21,30.86 144.4,30.86 145.29,31.88 149.61,31.88 149.61,26.67 149.1,26.29 145.54,26.29 145.54,25.65 143.38,25.65 C23.2 | 133.1,36.07 130.44,36.07 S3.1 128.15,34.16 121.41,34.16 v120.65,33.4 120.52,33.27 v116.59,33.27 v115.44,33.27 v114.3,33.27 | S5.1 132.62,50.26 133.1,50.04 | 133.1,50.04 133.1,36.07 | R49.E 71.5,75.82 67.31,80.01 57.66,80.01 56.64,81.03 43.69,81.03 35.3,72.64 DIS1.1 | SL1.1 67.69,5.08 67.69,6.99 67.44,7.24 67.56,7.24 | 67.56,7.24 67.56,16.38 67.61,23.23 67.56,26.67 61.72,29.84 | 61.72,29.84 61.72,33.53 61.72,36.32 61.72,40.13 61.47,55.88 61.47,72.14 63.5,74.17 71.63,74.17 71.63,74.93 71.37,75.18 | C20.- 162.09,30.95 163.19,29.97 163.19,21.84 164.85,21.84 TR1.2 164.85,14.22 160.53,14.22 159.77,13.46 | 159.51,2.03 160.78,1.02 178.56,1.02 178.56,1.27 178.82,1.52 197.1,1.52 197.17,1.46 C5.- 199.9,4.06 202.95,7.11 202.95,13.97 209.04,13.97 209.04,24.64 | 159.51,2.03 155.96,1.14 114.05,1.27 106.81,1.27 67.82,1.27 67.56,1.52 67.56,7.24 | 159.51,2.03 159.77,2.29 159.77,13.46 | 159.77,13.46 149.74,13.46 C24.2 | J1.1 209.04,30.28 209.04,24.64 | 209.04,24.64 208.79,24.38 D5.2 | 142.75,60.2 147.07,60.2 147.19,61.34 147.57,63.25 147.83,63.5 150.88,64.52 152.23,64.85 C12.2 | 61.72,29.84 61.72,28.96
N$138  (via drill 0.6)
  Top 0.406: v72.77,47.75 69.72,47.75 69.6,47.62 69.6,44.96 70.87,43.69 70.87,33.78 71.37,33.27 73.91,33.27 74.42,32.77 74.42,21.08 74.8,20.7 92.71,20.7 93.34,20.07 93.34,12.06 93.47,11.81 v93.47,11.68 | K1.1 157.35,4.32 158.62,5.59 158.62,10.03 168.91,10.03 | 168.91,10.03 169.42,10.03 170.43,9.02 170.43,3.56 172.34,1.65 179.58,1.65 179.58,15.49 178.69,16.38 v178.69,20.83 179.32,20.7 183.9,20.7 184.02,20.83 184.02,28.45 184.15,28.57 v190.75,28.57 | v96.27,11.68 96.14,11.81 96.14,19.3 96.27,19.43 104.65,19.43 105.16,18.92 v105.16,18.41 111.12,18.41 115.82,13.72 128.78,13.72 129.16,14.1 133.73,14.1 133.86,13.97 139.32,13.97 139.83,13.59 166.12,13.59 v167.39,14.86 | v169.16,8.89 169.42,9.91 168.91,10.03
  Bottom 0.406: C15.1 186.56,31.88 186.18,31.88 186.26,31.8 R13.2 186.26,28.91 186.31,29.46 190.37,29.46 v190.75,28.57 | IC7.35 76.35,58.4 76.33,58.42 74.17,58.42 72.52,56.77 72.52,48.01 v72.77,47.75 | R10.2 180.31,22.07 179.71,21.08 179.71,20.7 | 179.71,20.7 179.71,18.52 T3.2 | v178.69,20.83 179.58,20.83 179.71,20.7 | C14.+ 101.98,19.05 104.52,19.05 v105.16,18.41 | v96.27,11.68 v93.47,11.68 | v167.39,14.86 167.39,10.16 167.89,9.65 v169.16,8.89
  Bottom 0.61: R10.2 R11.2 180.26,26.72 R16.2
N$139
  Bottom 0.406: L2.1 146.66,28.2
  Bottom 1.016: Q12.3 144.53,6.86 144.53,8.13 123.44,8.13 123.44,15.49 131.7,15.49 132.72,16.51 132.72,20.07 132.21,20.19 117.86,20.19 117.86,20.95 116.33,21.84
  Bottom 1.27: L2.1 145.16,28.19 C23.1 141.73,28.2 137.16,29.59 116.33,29.59 116.33,21.84 117.6,20.95 117.73,20.83 C21.+
N$140  (via drill 0.6)
  Top 0.406: K1.3 135.13,8.51 134.37,9.27 98.81,9.27 97.92,10.16 97.92,16 97.54,16.38 97.54,18.16 97.92,18.54 102.23,18.54 102.87,17.91 102.87,16.26 103.25,15.88 109.73,15.88 v110.24,15.37 | v190.75,13.84 190.75,12.06 189.74,11.05 189.74,7.11 188.72,6.1 v188.72,4.19
  Top 0.61: T2.2 172.47,5.71 172.47,9.4 170.43,11.43 156.97,11.43 153.92,8.38 137.92,8.38 v137.92,4.32 137.92,1.4 78.74,1.4 SL1.3
  Bottom 0.406: SL1.3 D19.A | K1.3 v137.92,4.32 | v110.24,15.37 110.24,16.08 D17.C | R19.2 176.07,11.38 178.69,8.76 178.69,5.46 178.56,5.33 | R8.2 v190.75,13.84 | v188.72,4.19 189.61,4.32 189.36,4.06
  Bottom 0.61: IC3.7 185.8,4.19 185.93,4.06
  Bottom 1.016: T2.2 176.53,5.33 178.56,5.33 180.85,5.33 182.12,4.06 185.93,4.06 189.36,4.06 C5.+ 191.96,4.63 192.02,6.86 198.37,6.86 200.15,8.64 200.15,14.22 199.9,14.48 199.63,14.73 198.09,16.53 | D5.1 198.09,16.53 | 198.09,16.53 R7.2
  Bottom 1.27: F1.1 195.58,27.15 D5.1
N$141  (via drill 0.6)
  Top 0.406: v127,24.64 127,20.07 118.75,20.07 116.71,23.37 116.71,30.48 116.59,30.61 109.73,30.61 109.73,23.62 106.05,23.62 105.28,24.51 v105.28,29.08
  Bottom 0.406: R28.1 106.43,29.34 106.3,29.21 105.28,29.21 | 105.28,29.21 103.3,29.21 R51.2 | Q1.2 130.19,24.64 v127,24.64 | v105.28,29.08 105.28,29.21
N$142  (via drill 0.6)
  Top 0.406: v85.6,74.17 84.33,73.91 v84.33,71.12 | v82.55,60.07 v82.55,62.74 | v86.61,29.59 86.61,40.01 74.55,40.01 v73.66,40.89
  Top 1.016: v85.6,74.17 87,73.28 107.31,73.28 JP1.1
  Bottom 0.406: PR1.2 PR1.3 v85.6,74.17 | v84.33,71.12 83.57,69.34 83.06,68.58 83.06,67.43 IC7.5 83.06,67.36 83.06,63.5 82.55,62.99 v82.55,62.74 | v82.55,60.07 81.79,60.71 81.7,60.8 IC7.38 77.73,60.83 74.55,60.83 74.54,60.83 69.22,60.83 69.22,43.43 73.91,43.43 | 73.91,43.43 74.68,43.43 | R51.1 v86.61,29.59 | v73.66,40.89 73.66,43.18 73.91,43.43 | 110.24,73.41 103.63,73.41 103.63,70.48 R40.1 103.5,70.41 103.5,68.96 103.38,68.83 100.84,68.83 99.95,69.72 99.57,70.23 98.3,70.23 98.04,69.98 98.04,62.87 92.46,62.87 91.19,61.59 IC7.17 | 110.36,73.41 110.24,73.41 | 110.24,73.41 JP1.1
  Bottom 0.61: C26.2 75.69,50.29 75.69,46.35 74.58,44.99 L3.1 74.58,43.53 74.68,43.43
N$143
  Bottom 0.406: Q8.1 81.27,31.43 R44.1 81.97,31.42 82.04,31.37 82.04,25.91 81.79,25.53 76.5,25.53 Q11.3
N$144  (via drill 0.6)
  Top 0.406: v143.76,45.97 143.76,50.8 138.18,50.8 138.18,57.28 120.4,57.28 112.65,64.9 94.49,64.77 v94.49,66.55
  Bottom 0.406: IC7.3 81.42,71.51 81.41,72.14 94.23,72.14 | 94.23,72.14 94.49,71.75 v94.49,66.55 | 94.23,72.14 94.49,71.88 94.49,75.69 95.25,76.71 95.25,77.98 95,78.23 90.93,78.23 90.93,77.22 PR1.7 | Q5.B 141.22,45.97 v143.76,45.97
N$145
  Top 0.406: X1.3 215.28,44.6 215.26,44.58 215.26,43.81 217.18,43.81 X1.2
N$146  (via drill 0.6)
  Top 0.406: 143.51,12.7 169.67,12.7 171.32,14.86 171.7,15.37 171.83,15.62 v175.51,15.62 | 143.51,12.7 v130.3,12.7 | v74.42,47.62 74.42,49.28 68.2,49.28 68.2,45.21 69.72,43.18 69.72,33.4 70.99,32.13 73.03,32.13 73.41,31.75 73.41,19.94 73.53,19.81 91.82,19.81 92.2,19.43 92.2,14.86 91.31,13.97 91.31,11.68 96.14,6.86 127.25,6.86 128.14,6.1 128.14,2.79 128.4,2.54 136.53,2.54 136.53,9.4 143.26,9.4 143.51,9.65 143.51,12.7
  Bottom 0.406: 130.43,12.83 132.08,12.83 132.41,13.01 R15.2 134.37,14.28 134.62,16.26 136.14,18.03 D11.A | 130.43,12.83 128.01,13.97 C31.1 | v130.3,12.7 130.18,12.83 130.43,12.83 | IC7.33 79.29,55.8 78.36,54.36 73.91,54.36 73.66,54.23 73.66,49.15 74.42,48.39 v74.42,47.62 | R19.1 v175.51,15.62
N$147  (via drill 0.6)
  Top 0.406: v92.84,66.29 92.84,64.64 93.98,64.01 112.14,64.01 120.02,56.39 123.7,56.39 v123.7,55.88 | v112.65,29.21 112.65,22.73 v81.53,22.73
  Bottom 0.406: IC7.9 86.22,70.6 86.36,70.61 93.09,70.61 93.09,66.93 v92.84,66.29 | v123.7,55.88 123.7,53.34 123.57,53.21 121.16,53.21 120.65,52.7 120.65,35.94 120.27,35.56 120.27,35.43 119.76,34.92 113.03,34.92 112.65,34.54 v112.65,29.21 | v81.53,22.73 79.38,22.73 77.28,22.73 Q11.1
N$148  (via drill 0.6)
  Top 0.406: v74.3,55.88 67.94,55.88 v67.82,55.75 | v68.33,42.04 64.14,42.04 v64.14,43.18
  Bottom 0.406: IC7.30 82.17,55.8 82.17,57.91 80.14,57.91 80.14,57.78 77.72,55.37 74.3,55.37 v74.3,55.88 | R55.1 v64.14,43.18 R56.2 | v67.82,55.75 67.82,42.55 v68.33,42.04
N$149  (via drill 0.6)
  Top 1.016: R49.A 62.61,79.88 57.91,75.18 28.45,75.18 27.69,74.42 27.69,70.61 27.43,70.36 24.13,70.36 DIS1.2
  Top 1.27: v71.75,30.48 67.94,26.67 26.16,26.67 25.53,26.04 25.53,13.72 24.26,12.45 15.88,12.45 16.13,12.7 16.13,20.57 13.46,23.24 11.43,23.24 11.43,36.2 12.7,37.47 16.38,37.47 18.92,40.01 v18.92,40.26 18.92,70.1 19.18,70.1 DIS1.2
  Bottom 0.61: R43.2 15.11,36.45 v18.92,40.26
  Bottom 0.813: DIS1.2 23.37,70.1 18.03,75.44 14.35,75.44 C29.1
  Bottom 1.016: R49.A 75.69,79.88 C32.1
  Bottom 1.27: Q8.3 v71.75,30.48
(copper drawn outside any net)
  shapes: Bottom area x177, Top area x52

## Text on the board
tNames: Reset | +400 | Kontrast | GM1- | GM1+ | Geiger Muller Counter 2014 | GM2- | GM2+ | Charge | GM3- | Masa | Power on | GM3+ | Power | E | +Acc | B | 2,4V (2x 1,2)
bNames: +400V | Spk | Mute | Disp light | LED | 2,5v | HV on | Speaker | prąd ładowania | +5V test | Disp. power | 1,24V | Masa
